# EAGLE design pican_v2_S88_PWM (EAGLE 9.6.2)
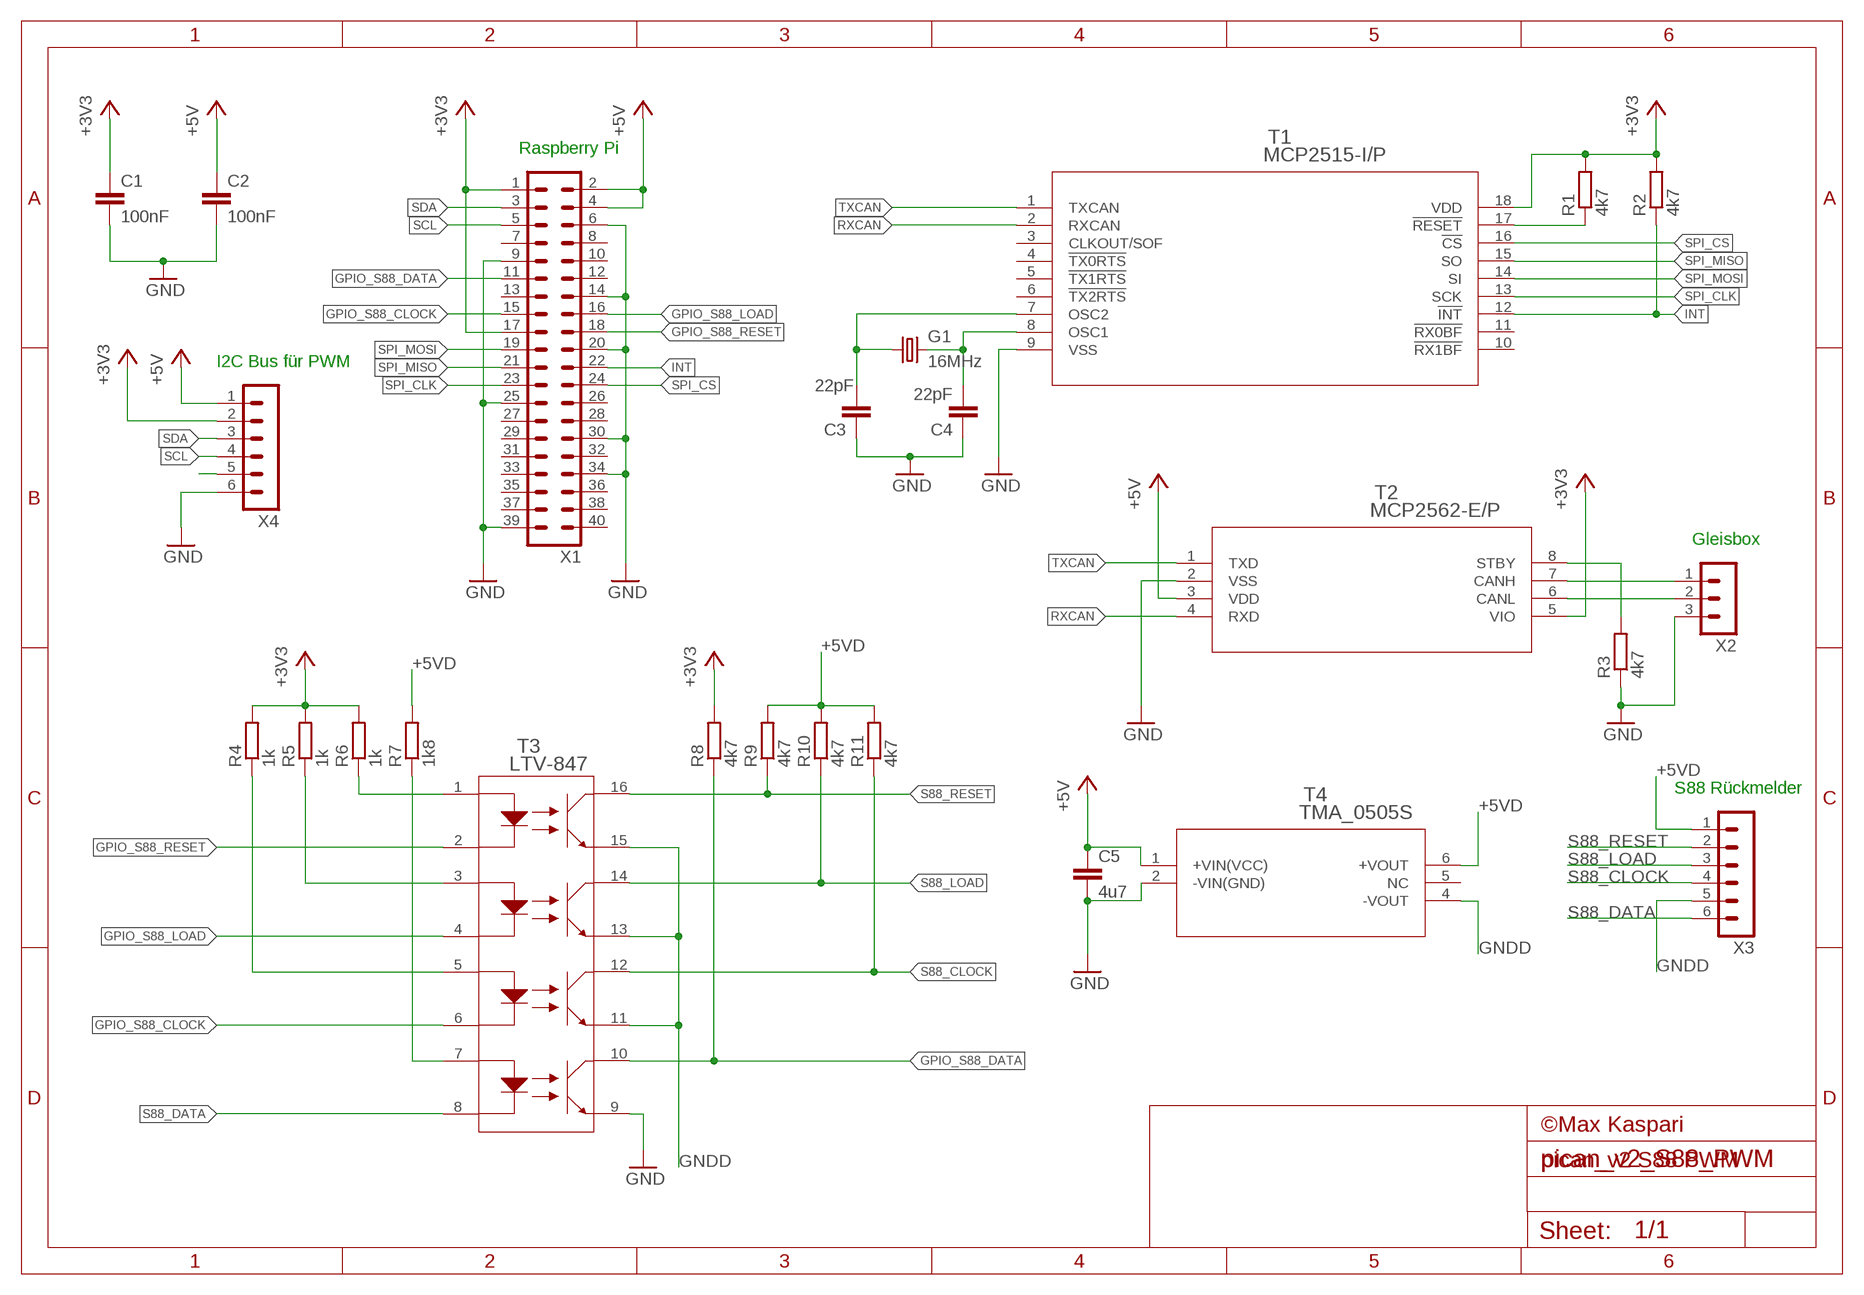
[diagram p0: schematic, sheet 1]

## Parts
C1  100nF  C-EU025-025X050  [C025-025X050]
C2  100nF  C-EU025-025X050  [C025-025X050]
C3  22pF  C-EU025-025X050  [C025-025X050]
C4  22pF  C-EU025-025X050  [C025-025X050]
C5  4u7  C-EUC1206  [C1206]
G1  16MHz  CRYSTALHC49S  [HC49/S]
R1  4k7  R-EU_0204/7  [0204/7]
R2  4k7  R-EU_0204/7  [0204/7]
R3  4k7  R-EU_0204/7  [0204/7]
R4  1k  R-EU_0204/7  [0204/7]
R5  1k  R-EU_0204/7  [0204/7]
R6  1k  R-EU_0204/7  [0204/7]
R7  1k8  R-EU_0204/7  [0204/7]
R8  4k7  R-EU_0204/7  [0204/7]
R9  4k7  R-EU_0204/7  [0204/7]
R10  4k7  R-EU_0204/7  [0204/7]
R11  4k7  R-EU_0204/7  [0204/7]
T1  MCP2515-I/P  [PDIP18_300MC_MCH]
T2  MCP2562-E/P  [PDIP8_300MC_MCH]
T3  LTV-847  [LTV-847_LTO]
T4  TMA_0505S  [TMA-1W-SINGLE]
X1  MA20-2  [MA20-2]
X2  MA03-1  [MA03-1_NUMBERTOP]
X3  MA06-1  [MA06-1_NUMBERTOP]
X4  MA06-1  [MA06-1_NUMBERTOP]

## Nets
+3V3: C1.1 R1.2 R2.2 R4.2 R5.2 R6.2 R8.2 T1.18(VDD) T2.5(VIO) X1.1 X1.17 X4.2
+5V: C2.1 C5.1 T2.3(VDD) T4.1(+VIN(VCC)) X1.2 X1.4 X4.1
+5VD: R7.2 R9.2 R10.2 R11.2 T4.6(+VOUT) X3.1
CANH: T2.7(CANH) X2.1
CANL: T2.6(CANL) X2.2
GND: C1.2 C2.2 C3.1 C4.1 C5.2 R3.1 T1.9(VSS) T2.2(VSS) T3.9 T4.2(-VIN(GND)) X1.6 X1.9 X1.14 X1.20 X1.25 X1.30 X1.34 X1.39 X2.3 X4.6
GNDD: T3.11 T3.13 T3.15 T4.4(-VOUT) X3.5
GPIO_S88_CLOCK: T3.6 X1.15
GPIO_S88_DATA: R8.1 T3.10 X1.11
GPIO_S88_LOAD: T3.4 X1.16
GPIO_S88_RESET: T3.2 X1.18
INT: R2.1 T1.12(!INT) X1.22
N$1: C4.2 G1.2 T1.8(OSC1)
N$2: C3.2 G1.1 T1.7(OSC2)
N$3: R1.1 T1.17(!RESET)
N$4: R3.2 T2.8(STBY)
N$10: R7.1 T3.7
N$11: R6.1 T3.1
N$12: R5.1 T3.3
N$13: R4.1 T3.5
N$15: X4.5
RXCAN: T1.2(RXCAN) T2.4(RXD)
S88_CLOCK: R11.1 T3.12 X3.4
S88_DATA: T3.8 X3.6
S88_LOAD: R10.1 T3.14 X3.3
S88_RESET: R9.1 T3.16 X3.2
SCL: X1.5 X4.4
SDA: X1.3 X4.3
SPI_CLK: T1.13(SCK) X1.23
SPI_CS: T1.16(!CS) X1.24
SPI_MISO: T1.15(SO) X1.21
SPI_MOSI: T1.14(SI) X1.19
TXCAN: T1.1(TXCAN) T2.1(TXD)
Unconnected: T1.3(CLKOUT/SOF) T1.4(!TX0RTS) T1.5(!TX1RTS) T1.6(!TX2RTS) T1.10(!RX1BF) T1.11(!RX0BF) T4.5(NC) X1.7 X1.8 X1.10 X1.12 X1.13 X1.26 X1.27 X1.28 X1.29 X1.31 X1.32 X1.33 X1.35 X1.36 X1.37 X1.38 X1.40

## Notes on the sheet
- Raspberry Pi
- I2C Bus für PWM
- Gleisbox
- S88 Rückmelder
- ©Max Kaspari
- pican_v2 S88 PWM

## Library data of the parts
C1-C5 = rcl:C-EU: CAPACITOR, European symbol; SPICEPREFIX: C
G1 = crystal:CRYSTAL: CRYSTAL; OC_FARNELL: 1667008; OC_NEWARK: unknown
R1-R11 = rcl:R-EU_: RESISTOR, European symbol; SPICEPREFIX: R
T1 = modellbahn:MCP2515-I/P; BUILT_BY: EMA_UL_Team; MANUFACTURER_PART_NUMBER: MCP2515-I/P; SOURCELIBRARY: Microchip_2011-04-01; VENDOR: Microchip
T2 = modellbahn:MCP2562-E/P; BUILT_BY: EMA_UL_Team; MANUFACTURER_PART_NUMBER: MCP2562-E/P; SOURCELIBRARY: Microchip_2014-11-20; VENDOR: Microchip
T3 = modellbahn:LTV-847; BUILT_BY: EMA_Cory; COPYRIGHT: Copyright (C) 2018 Accelerated Designs. All rights reserved; DATASHEET: https://media.digikey.com/pdf/Data%20Sheets/Lite-On%20PDFs/LTV-817_827_847(M,S,S_TA1).pdf; MANUFACTURER_PART_NUMBER: LTV-847; SOURCELIBRARY: Add_to_database_2020-10-26; VENDOR: Lite-On
T4 = modellbahn:TMA_0505S; BUILT_BY: EMA_Justin; COPYRIGHT: Copyright (C) 2018 Accelerated Designs. All rights reserved; DATASHEET: https://www.tracopower.com/products/tma.pdf; MANUFACTURER_PART_NUMBER: TMA 0505S; SOURCELIBRARY: Traco_Power_2020-05-29; VENDOR: Traco Power
X1 = con-lstb:MA20-2: PIN HEADER; OC_FARNELL: unknown; OC_NEWARK: unknown
X2 = modellbahn:MA03-1: PIN HEADER; OC_FARNELL: unknown; OC_NEWARK: unknown
X3 X4 = modellbahn:MA06-1: PIN HEADER; OC_FARNELL: unknown; OC_NEWARK: unknown

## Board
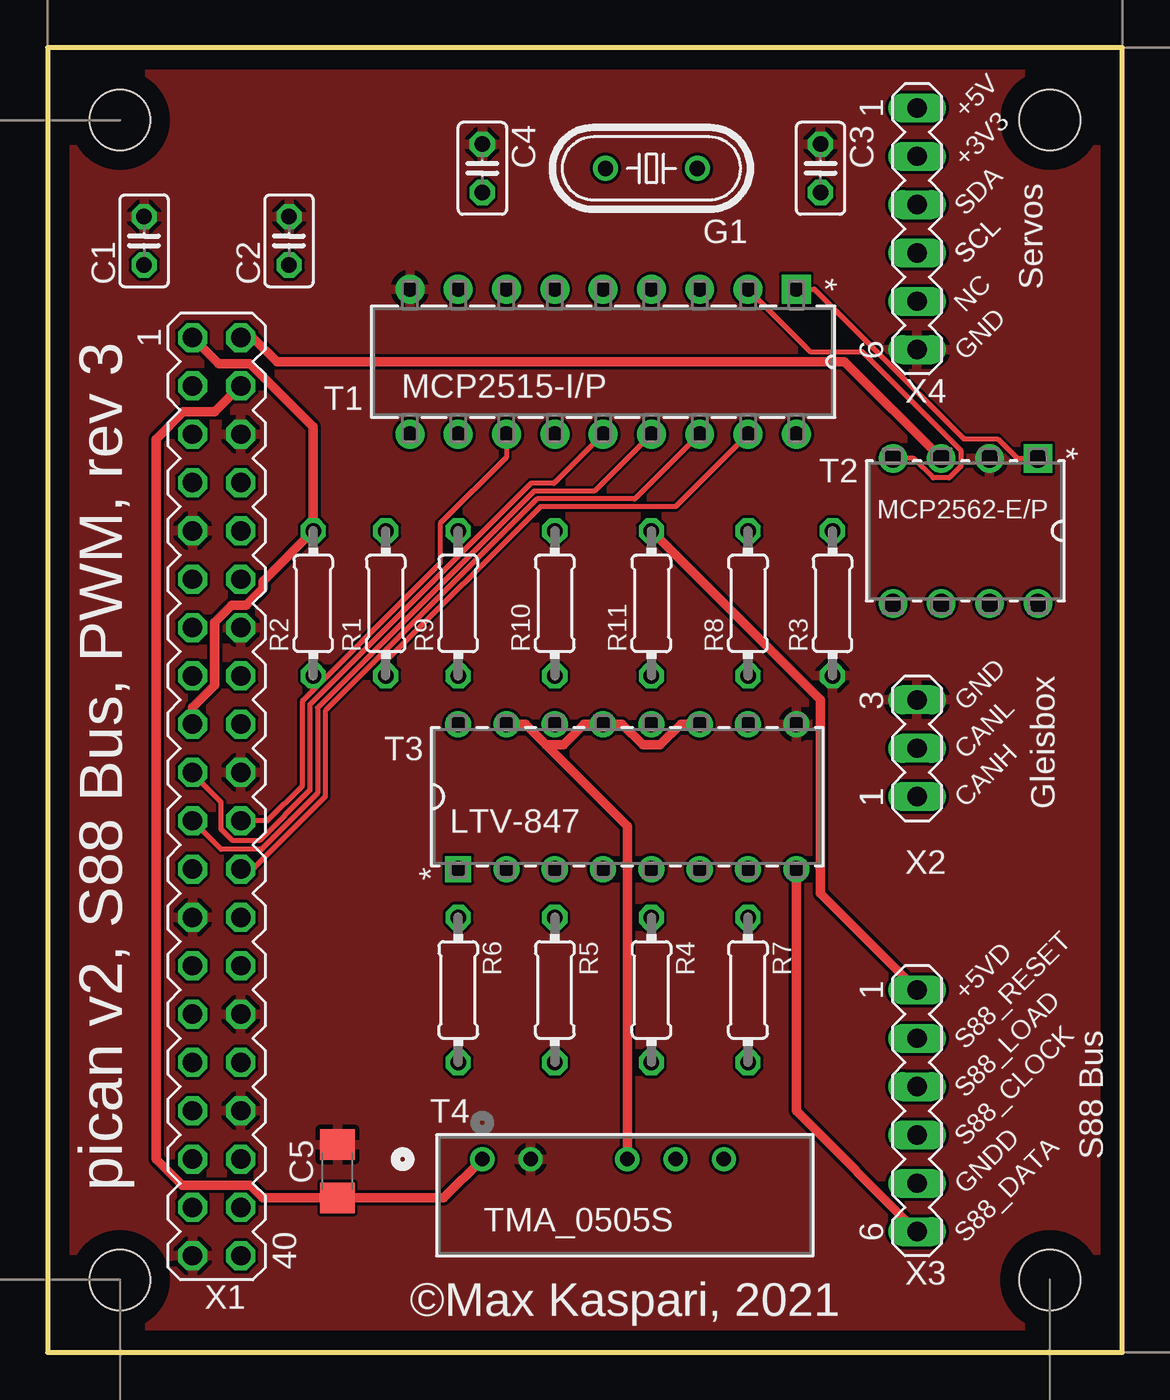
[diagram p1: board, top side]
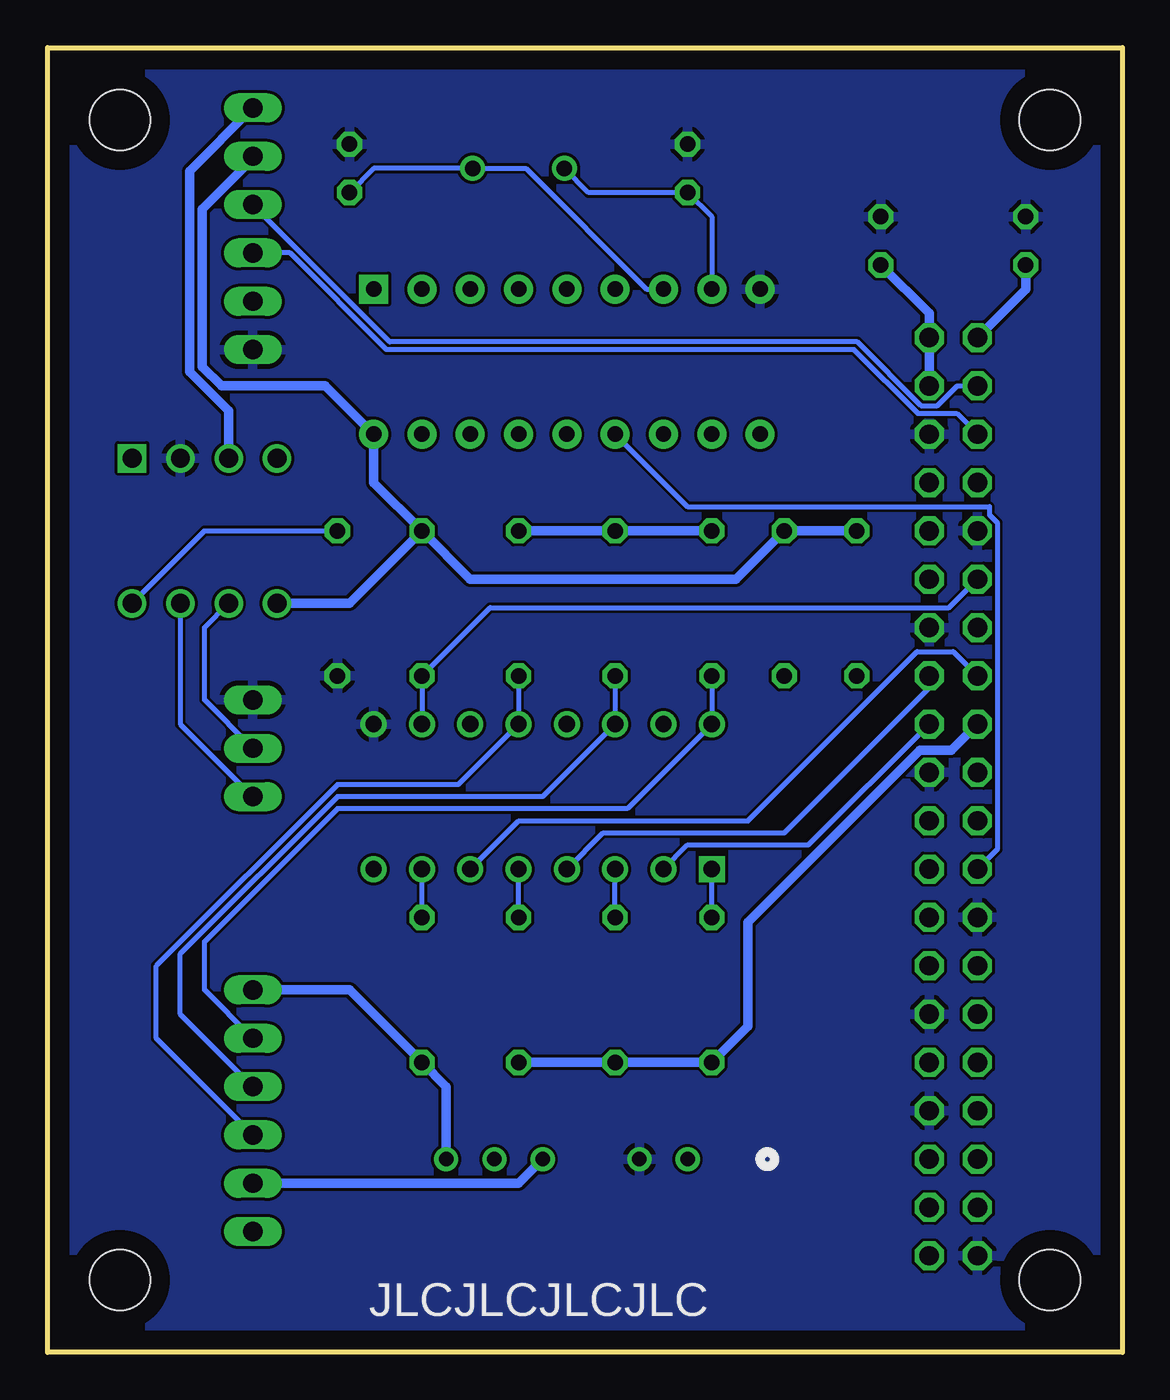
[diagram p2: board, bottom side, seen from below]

Size 56.52 x 68.58 mm. Coordinates in mm from the lower left corner, seen from the top.
Outline: 0,0 56.52,0 56.52,68.58 0,68.58 0,0
Copper layers (1*16): Top 0.035mm / dielectric 1.5mm / Bottom 0.035mm
Design rules "default *": minimum track width 6mil, minimum drill 0.35mm, track to track 6mil, track to pad 6mil, pad to pad 6mil, via to via 6mil, smd to smd 6mil, copper to edge 40mil, drill to drill 6mil, minimum pad ring 10mil, minimum via ring 8mil, stop-mask expansion 4mil, vias tented up to drill 0mil, thermal gap 10mil

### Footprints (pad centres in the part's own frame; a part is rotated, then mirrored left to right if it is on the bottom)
C025-025X050 = drill 0.813 octagon: 1 -1.27,0; 2 1.27,0
C1206 = smd 1.6 x 1.8: 1 -1.4,0; 2 1.4,0
HC49/S = drill 0.813: 1 -2.413,0; 2 2.413,0
0204/7 = drill 0.813 octagon: 1 -3.81,0; 2 3.81,0
PDIP18_300MC_MCH = drill 0.813 pad 1.524 square: 1 -3.81,10.16 | drill 0.813 pad 1.524: 2 -3.81,7.62; 3 -3.81,5.08; 4 -3.81,2.54; 5 -3.81,0; 6 -3.81,-2.54; 7 -3.81,-5.08; 8 -3.81,-7.62; 9 -3.81,-10.16; 10 3.81,-10.16; 11 3.81,-7.62; 12 3.81,-5.08; 13 3.81,-2.54; 14 3.81,0; 15 3.81,2.54; 16 3.81,5.08; 17 3.81,7.62; 18 3.81,10.16
PDIP8_300MC_MCH = drill 0.991 pad 1.499 square: 1 -3.81,3.81 | drill 0.991 pad 1.499: 2 -3.81,1.27; 3 -3.81,-1.27; 4 -3.81,-3.81; 5 3.81,-3.81; 6 3.81,-1.27; 7 3.81,1.27; 8 3.81,3.81
LTV-847_LTO = drill 0.864 pad 1.372 square: 1 -3.81,8.89 | drill 0.864 pad 1.372: 2 -3.81,6.35; 3 -3.81,3.81; 4 -3.81,1.27; 5 -3.81,-1.27; 6 -3.81,-3.81; 7 -3.81,-6.35; 8 -3.81,-8.89; 9 3.81,-8.89; 10 3.81,-6.35; 11 3.81,-3.81; 12 3.81,-1.27; 13 3.81,1.27; 14 3.81,3.81; 15 3.81,6.35; 16 3.81,8.89
TMA-1W-SINGLE = drill 0.762 pad 1.27: 1 0,0; 2 2.54,0; 4 7.62,0; 5 10.16,0; 6 12.7,0
M3HOLE = hole 3.2: 0,0
MA20-2 = drill 1.016 octagon: 1 -24.13,-1.27; 2 -24.13,1.27; 3 -21.59,-1.27; 4 -21.59,1.27; 5 -19.05,-1.27; 6 -19.05,1.27; 7 -16.51,-1.27; 8 -16.51,1.27; 9 -13.97,-1.27; 10 -13.97,1.27; 11 -11.43,-1.27; 12 -11.43,1.27; 13 -8.89,-1.27; 14 -8.89,1.27; 15 -6.35,-1.27; 16 -6.35,1.27; 17 -3.81,-1.27; 18 -3.81,1.27; 19 -1.27,-1.27; 20 -1.27,1.27; 21 1.27,-1.27; 22 1.27,1.27; 23 3.81,-1.27; 24 3.81,1.27; 25 6.35,-1.27; 26 6.35,1.27; 27 8.89,-1.27; 28 8.89,1.27; 29 11.43,-1.27; 30 11.43,1.27; 31 13.97,-1.27; 32 13.97,1.27; 33 16.51,-1.27; 34 16.51,1.27; 35 19.05,-1.27; 36 19.05,1.27; 37 21.59,-1.27; 38 21.59,1.27; 39 24.13,-1.27; 40 24.13,1.27
MA03-1_NUMBERTOP = drill 1.016 long: 1 -2.54,0; 2 0,0; 3 2.54,0
MA06-1_NUMBERTOP = drill 1.016 long: 1 -6.35,0; 2 -3.81,0; 3 -1.27,0; 4 1.27,0; 5 3.81,0; 6 6.35,0

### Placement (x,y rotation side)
C1  5.08,58.42 90 top
C2  12.7,58.42 90 top
C3  40.64,62.23 270 top
C4  22.86,62.23 270 top
C5  15.24,9.53 90 top
G1  31.75,62.23 180 top
R1  17.78,39.37 90 top
R2  13.97,39.37 90 top
R3  41.27,39.37 90 top
R4  31.75,19.05 270 top
R5  26.67,19.05 270 top
R6  21.59,19.05 270 top
R7  36.83,19.05 270 top
R8  36.83,39.37 90 top
R9  21.59,39.37 90 top
R10  26.67,39.37 90 top
R11  31.75,39.37 90 top
T1  29.21,52.07 270 top
T2  48.26,43.18 270 top
T3  30.48,29.21 90 top
T4  22.86,10.16 0 top
U$1  [M3HOLE]  3.81,64.77 0 top
U$2  [M3HOLE]  3.81,3.81 0 top
U$3  [M3HOLE]  52.7,3.81 0 top
U$4  [M3HOLE]  52.7,64.77 0 top
X1  8.89,29.21 270 top
X2  45.72,31.75 90 top
X3  45.72,12.7 270 top
X4  45.72,59.05 270 top

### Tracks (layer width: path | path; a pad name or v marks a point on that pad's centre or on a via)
+3V3
  Top 0.508: X1.1 8.99,51.97 10.64,51.97 13.97,48.64 R2.2 11.33,40.54 11.33,40.16 10.44,39.27 9.68,39.27 8.79,38.38 8.79,35.08 7.62,33.91 X1.17
  Bottom 0.508: X1.1 5.08,55.88 C1.1 | R2.2 R1.2 20.32,40.64 34.29,40.64 R8.2 | R8.2 39.37,45.72 T1.18 41.91,50.8 47.37,50.8 48.39,51.82 48.39,60.07 45.72,62.74 X4.2 | R8.2 40.64,39.37 T2.5 | X1.17 8.99,31.65 10.64,31.65 19.68,22.61 19.68,17.14 R6.2 R5.2 R4.2
+5V
  Top 0.508: X1.2 10.79,53.34 12.06,52.07 41.91,52.07 T2.3 | T4.1 20.82,8.12 C5.1 11.31,8.12 10.64,8.79 7.09,8.79 5.71,10.16 5.71,48.01 7.14,49.43 8.79,49.43 X1.4
  Bottom 0.508: C2.1 10.16,54.61 X1.2 X1.4 | T2.3 46.99,49.48 49.05,51.54 49.05,62.08 X4.1
+5VD
  Top 0.508: R11.2 40.64,34.29 40.64,24.13 X3.1
  Bottom 0.508: T4.6 35.56,13.97 R7.2 40.64,19.05 X3.1 | R9.2 R10.2 R11.2
CANH
  Bottom 0.254: T2.7 49.53,33.02 X2.1
CANL
  Bottom 0.254: X2.2 48.26,34.29 48.26,38.1 T2.6
GND
  pour Bottom: 0,68.58 0,0 56.52,0 56.52,68.58
  pour Top: 0,68.58 56.52,68.58 56.52,0 0,0
GNDD
  Top 0.508: 26.22,31.93 27.12,31.93 28.21,33.02 T3.13 30.2,33.02 31.3,31.93 32.2,31.93 33.3,33.02 T3.11 | T3.15 25.12,33.02 26.22,31.93 | T4.4 30.48,27.66 26.22,31.93
  Bottom 0.508: T4.4 31.75,8.89 X3.5
GPIO_S88_CLOCK
  Bottom 0.254: T3.6 31.75,27.94 19.68,27.94 10.79,36.83 8.89,36.83 X1.15
GPIO_S88_DATA
  Bottom 0.254: T3.10 R8.1 33.25,39.14 9.12,39.14 X1.11
GPIO_S88_LOAD
  Bottom 0.254: T3.4 27.3,27.3 17.78,27.3 10.16,34.92 X1.16
GPIO_S88_RESET
  Bottom 0.254: T3.2 22.86,26.67 16.51,26.67 X1.18
INT
  Top 0.254: 13.97,34.8 R2.1 | 13.97,34.8 13.39,34.22 13.39,29.77 11.56,27.94 X1.22 | T1.12 24.13,47.05 20.65,43.57 20.65,41.48 13.97,34.8
N$1
  Bottom 0.254: T1.8 21.59,59.69 C4.2 28.07,60.96 G1.2
N$2
  Bottom 0.254: C3.2 39.37,62.23 G1.1 31.37,62.23 25.02,55.88 T1.7
N$3
  Top 0.254: T1.17 33.02,44.45 25.92,44.45 17.78,36.31 R1.1
N$4
  Bottom 0.254: T2.8 48.26,43.18 R3.2
N$10
  Bottom 0.254: R7.1 T3.7
N$11
  Bottom 0.254: R6.1 T3.1
N$12
  Bottom 0.254: R5.1 T3.3
N$13
  Bottom 0.254: R4.1 T3.5
RXCAN
  Top 0.254: T1.2 40.11,52.6 42.83,52.6 48.02,47.42 48.02,46.56 47.42,45.96 46.56,45.96 45.53,46.99 T2.4
S88_CLOCK
  Bottom 0.254: R11.1 T3.12 34.92,29.84 41.27,29.84 50.8,20.32 50.8,16.51 X3.4
S88_DATA
  Top 0.508: T3.8 39.37,12.7 X3.6
S88_LOAD
  Bottom 0.254: R10.1 T3.14 30.48,29.21 41.27,29.21 49.53,20.95 49.53,17.78 X3.3
S88_RESET
  Bottom 0.254: R9.1 T3.16 26.04,28.57 41.27,28.57 48.26,21.59 48.26,19.05 X3.2
SCL
  Bottom 0.254: X1.5 8.71,49.35 10.76,49.35 14.11,52.7 38.69,52.7 43.77,57.78 X4.4
SDA
  Bottom 0.254: X1.3 8.69,50.8 9.73,49.76 10.59,49.76 13.94,53.11 38.52,53.11 40.41,55 40.41,55.02 X4.3
SPI_CLK
  Bottom 0.254: T1.13 22.86,44.45 6.99,44.45 6.99,44.02 6.58,43.61 6.58,26.44 X1.23
SPI_CS
  Top 0.254: T1.16 30.89,44.86 25.75,44.86 14.61,33.71 14.61,29.21 10.79,25.4 X1.24
SPI_MISO
  Top 0.254: T1.15 28.75,45.26 25.58,45.26 19.05,38.73 14.2,33.88 14.2,29.38 11.26,26.44 9.12,26.44 X1.21
SPI_MOSI
  Top 0.254: T1.14 26.62,45.67 25.41,45.67 13.79,34.05 13.79,29.55 11.14,26.9 9.73,26.9 9.12,27.51 9.12,28.92 7.62,30.42 X1.19
TXCAN
  Top 0.254: T1.1 40.31,55.88 48.17,48.02 49.96,48.02 50.98,46.99 T2.1

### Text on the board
tPlace: NC | S88_DATA
tNames: +5V | +3V3 | SDA | SCL | SCL | Servos | GND | GND | CANL | CANH | Gleisbox | +5VD | S88_RESET | S88_LOAD | S88_CLOCK | S88 Bus | pican v2, S88 Bus, PWM, rev 3 | GNDD | ©Max Kaspari, 2021
bNames: JLCJLCJLCJLC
